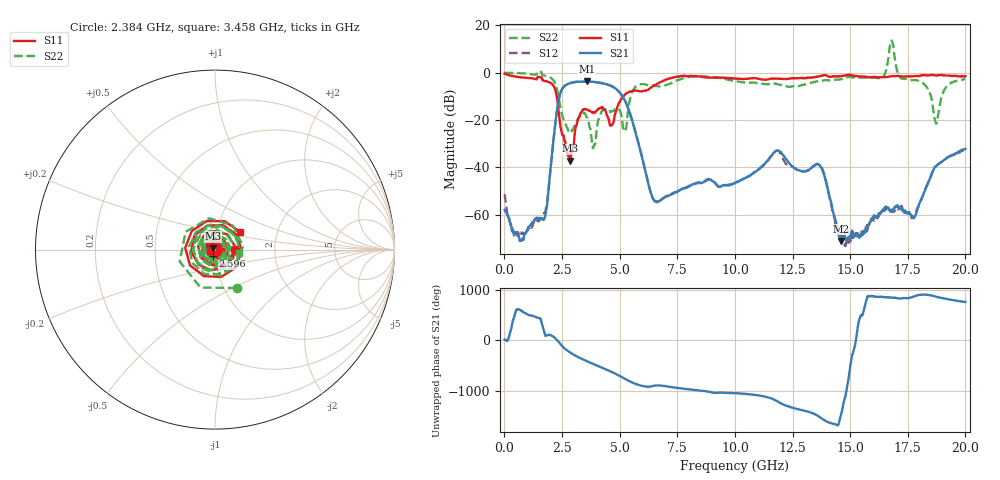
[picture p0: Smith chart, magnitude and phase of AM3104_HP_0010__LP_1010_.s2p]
!Created with skrf (http://scikit-rf.org).
# Hz S RI R 50.0
!freq ReS11 ImS11 ReS21 ImS21 ReS12 ImS12 ReS22 ImS22
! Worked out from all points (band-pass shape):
!   1601 points, 10 MHz to 20 GHz, reference 50 ohm
!   highest |S21| = -3.69 dB at 3.571 GHz (marker M1); lowest = -71.1 dB at 14.6 GHz (marker M2)
!   |S21| within 3 dB of the highest: 2.516 GHz to 4.831 GHz (2.315 GHz wide, 63 % of centre)
!   lowest |S11| = -37.2 dB at 2.859 GHz (marker M3), VSWR 1.03, Z = 48.9 + j0.769 ohm
!   |S11| at or under -10 dB: 2.272 GHz to 5.157 GHz (2.885 GHz wide, 77.7 % of centre)
!   |S22| runs from -31.8 to 13.6 dB; largest |S21 - S12| = 0.052
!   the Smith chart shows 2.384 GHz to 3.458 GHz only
!   S11 on the Smith chart (normalised r, x): 2.384 GHz: 1.25, -0.01; 2.596 GHz: 0.97, -0.07; 3.458 GHz: 1.29, +0.27
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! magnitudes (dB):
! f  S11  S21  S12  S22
! 10 MHz  -0.4  -57.9  -51.3  0.0
! 472.3 MHz  -1.6  -67.8  -68.5  -0.1
! 1.722 GHz  -3.4  -62.1  -59.3  -1.2
! 2.384 GHz  -18.9  -10.2  -10.3  -12.2
! 2.596 GHz  -28.2  -5.7  -5.7  -20.5
! 2.859 GHz  -37.2  -4.3  -4.4  -25.2
! 3.346 GHz  -16.5  -3.8  -3.8  -16.9
! 3.458 GHz  -15.4  -3.7  -3.7  -17.2
! 3.571 GHz  -15.5  -3.7  -3.8  -18.8
! 3.871 GHz  -16.7  -3.8  -3.8  -31.3
! 4.295 GHz  -15.1  -4.5  -4.5  -15.7
! 5.157 GHz  -10.0  -10.5  -10.5  -23.6
! 5.695 GHz  -7.5  -25.3  -25.3  -5.9
! 6.682 GHz  -4.4  -54.4  -54.2  -5.7
! 10.01 GHz  -2.5  -46.7  -46.6  -3.6
! 11.83 GHz  -2.5  -32.9  -33.0  -4.8
! 13.34 GHz  -2.1  -40.1  -40.1  -4.2
! 14.6 GHz  -1.5  -71.1  -69.5  -2.7
! 16.68 GHz  -1.6  -57.4  -58.0  7.3
! 17.79 GHz  -1.4  -61.1  -60.9  -3.0
! 18.73 GHz  -1.2  -39.4  -39.5  -21.4
! 20 GHz  -1.4  -32.2  -31.8  -2.6
